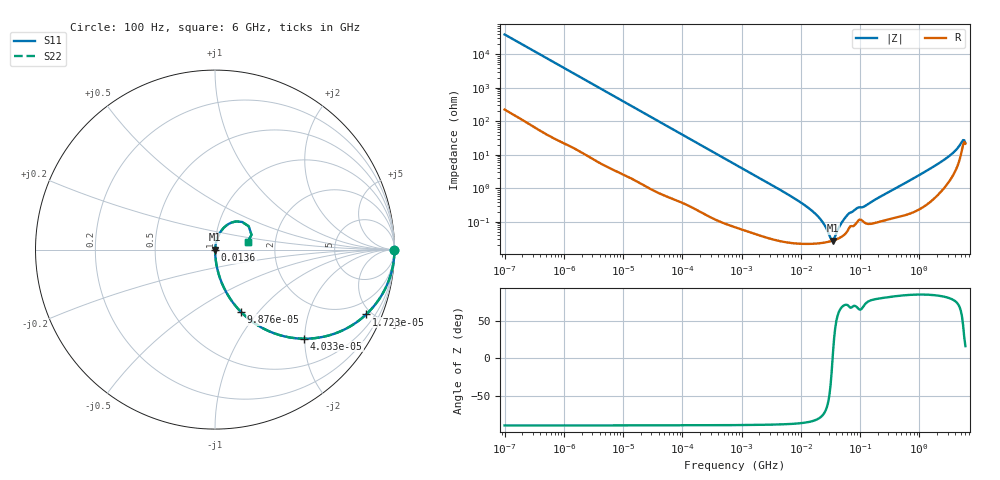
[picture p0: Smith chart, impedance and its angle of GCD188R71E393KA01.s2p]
!Murata Part Number: GCD188R71E393KA01
!These Parameters are Measured in Series Mode Connection
!Data Generated on Jan 08, 2026
!  o--ll--o
!Port1  Port2
!  o------o
!Operation Temp=25[degC], DC Bias Voltage=0[V]
!Freq. Start=100[Hz] Stop=6[GHz] 401[Steps]
# Hz S RI R 50
!Freq.(Hz) S11(Real) S11(Imag) S21(Real) S21(Imag) S12(Real) S12(Imag) S22(Real) S22(Imag)
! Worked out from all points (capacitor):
!   401 points, 100 Hz to 6 GHz, reference 50 ohm
!   read as one part in series: C = 40.4 nF near 109 Hz
!   lowest |Z| = 28 mohm at 34.83 MHz (marker M1)
!   series resonance near 34.43 MHz, so ESL is about 530 pH
!   S11 on the Smith chart (normalised r, x): 100 Hz: open; 17.23 kHz: 1.03, -4.65; 40.34 kHz: 1.01, -1.99; 98.76 kHz: 1.01, -0.82; 13.6 MHz: 1.00, -0.01; 6 GHz: 1.44, +0.12
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100  1 -0.00254  2.11e-05 0.00254  2.11e-05 0.00254  1 -0.00254
2008  0.9972 -0.0504  0.00285 0.0504  0.00285 0.0504  0.9972 -0.0504
7695  0.9631 -0.1854  0.0369 0.1854  0.0369 0.1854  0.9631 -0.1854
17227  0.8422 -0.3611  0.1578 0.3611  0.1578 0.3611  0.8422 -0.3611
40335  0.4983 -0.4964  0.5017 0.4964  0.5017 0.4964  0.4983 -0.4964
98762  0.1455 -0.348  0.8545 0.348  0.8545 0.348  0.1455 -0.348
264476  0.0245 -0.1496  0.9755 0.1496  0.9755 0.1496  0.0245 -0.1496
774597  0.00346 -0.0525  0.9965 0.0525  0.9965 0.0525  0.00346 -0.0525
5809218  0.000293 -0.00692  0.9997 0.00692  0.9997 0.00692  0.000293 -0.00692
1.360128e7  0.000228 -0.00257  0.9998 0.00257  0.9998 0.00257  0.000228 -0.00257
1.555665e7  0.000227 -0.00212  0.9998 0.00212  0.9998 0.00212  0.000227 -0.00212
2.225763e7  0.000236 -0.00109  0.9998 0.00109  0.9998 0.00109  0.000236 -0.00109
3.184506e7  0.000266 -0.000189  0.9997 0.000189  0.9997 0.000189  0.000266 -0.000189
3.482834e7  0.000278 2.85e-05  0.9997 -2.85e-05  0.9997 -2.85e-05  0.000278 2.85e-05
4.983056e7  0.000371 0.000931  0.9996 -0.000931  0.9996 -0.000931  0.000371 0.000931
6.518806e7  0.000656 0.00168  0.9993 -0.00168  0.9993 -0.00168  0.000656 0.00168
3.124326e8  0.00127 0.00789  0.9987 -0.00789  0.9987 -0.00789  0.00127 0.00789
1.431855e9  0.00488 0.0359  0.9951 -0.0359  0.9951 -0.0359  0.00488 0.0359
3.205649e9  0.024 0.0877  0.976 -0.0877  0.976 -0.0877  0.024 0.0877
4.385646e9  0.0626 0.1339  0.9374 -0.1339  0.9374 -0.1339  0.0626 0.1339
5.245841e9  0.1509 0.1541  0.8491 -0.1541  0.8491 -0.1541  0.1509 0.1541
6e9  0.1814 0.0418  0.8186 -0.0418  0.8186 -0.0418  0.1814 0.0418
